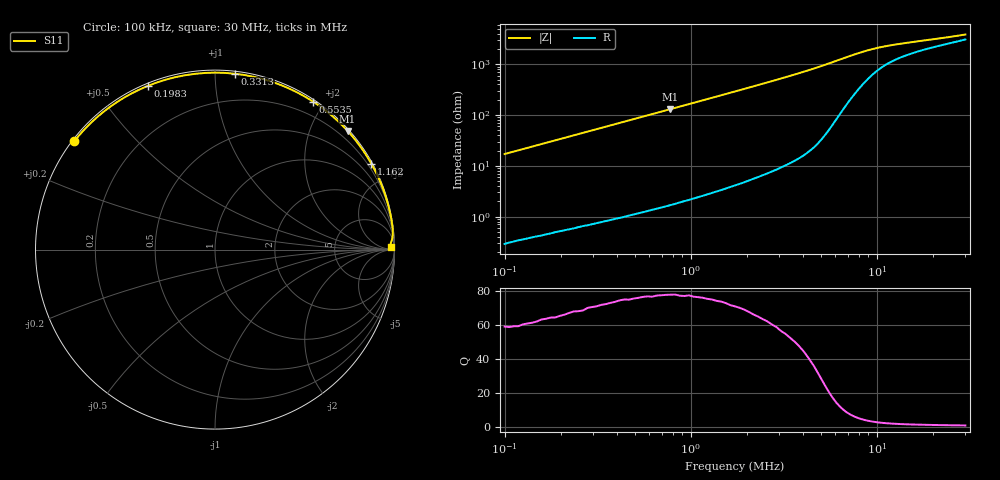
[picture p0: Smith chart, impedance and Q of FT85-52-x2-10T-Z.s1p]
! ListType=Log
!!FT85-52 x2 10T Z
# MHz S RI R 50
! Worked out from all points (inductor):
!   101 points, 100 kHz to 30 MHz, reference 50 ohm
!   read as one part to ground: L = 27.1 uH near 100 kHz
!   highest Q = 77.7 at 779.4 kHz (marker M1), where L = 26.7 uH
!   S11 on the Smith chart (normalised r, x): 100 kHz: 0.01, +0.34; 198.3 kHz: 0.01, +0.67; 331.3 kHz: 0.02, +1.12; 553.5 kHz: 0.02, +1.86; 1.162 MHz: 0.05, +3.90; 30 MHz: 62, +46
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0.1  -0.7831 0.6052
0.1186625  -0.7105 0.687
0.140808  -0.6188 0.7694
0.1670863  -0.506 0.8469
0.1982689  -0.3722 0.9129
0.2099064  -0.3234 0.9312
0.2352709  -0.2206 0.9607
0.2637003  -0.1124 0.9792
0.295565  -0.00142 0.9859
0.3312802  0.1097 0.9801
0.3713111  0.2182 0.9623
0.4406071  0.3708 0.9154
0.4938487  0.4631 0.8732
0.5535239  0.5462 0.8247
0.6568255  0.653 0.7445
0.7794058  0.7389 0.6611
0.8735868  0.7854 0.6061
0.9791484  0.8245 0.553
1.161882  0.8711 0.4782
1.459644  0.9153 0.3895
1.833715  0.9446 0.3141
2.582017  0.9708 0.2242
3.635686  0.9844 0.1569
5.41982  0.9907 0.0982
7.631539  0.9874 0.0622
10.15005  0.982 0.0434
15.13097  0.9779 0.0292
30  0.9794 0.0152
